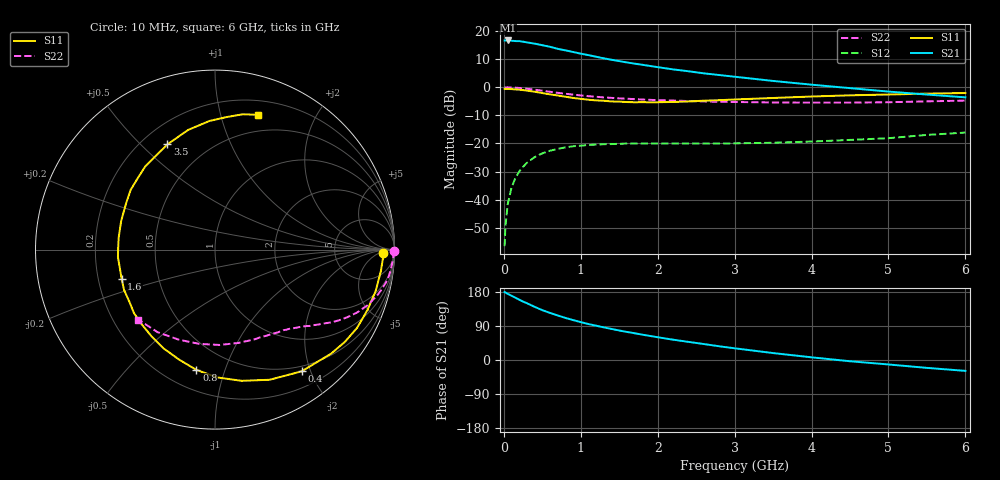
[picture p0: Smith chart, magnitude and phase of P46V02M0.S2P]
! SIEMENS Small Signal Semiconductors
! BFP182
! Si NPN RF Bipolar Junction Transistor in SOT143
! VCE = 6 V  IC = 2 mA
! Common Emitter S-Parameters:  March  1996
# GHz  S  MA  R  50
!  f  S11  S21  S12  S22
! GHz  MAG  ANG  MAG  ANG  MAG  ANG  MAG  ANG
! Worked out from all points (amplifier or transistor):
!   36 points, 10 MHz to 6 GHz, reference 50 ohm
!   highest |S21| = 16.6 dB at 50 MHz (marker M1)
!   |S21| within 3 dB of that: start of sweep to 704.2 MHz
!   unconditionally stable (mu >= 1): 2.231 GHz to 5.925 GHz
!   at 250 MHz: K = 0.12, MSG = 22.2 dB, |S12| = -28.3 dB
!   at 1.4 GHz: K = 0.66, MSG = 15.0 dB, |S12| = -20.2 dB
!   at 6 GHz: K = 0.99, MSG = 6.3 dB, |S12| = -16.1 dB
!   lowest NFmin = 1.10 dB at 450 MHz
!   S11 on the Smith chart (normalised r, x): 10 MHz: 27, -8; 400 MHz: 0.42, -1.86; 800 MHz: 0.32, -0.80; 1.6 GHz: 0.30, -0.14; 3.5 GHz: 0.30, +0.60; 6 GHz: 0.33, +1.32
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0.01  0.9351 -1.2  6.766 179.2  0.0015 88.4  0.9949 -0.5
0.02  0.9367 -3.2  6.755 178.4  0.0033 88.6  0.9911 -1.0
0.05  0.9318 -7.4  6.768 174.7  0.0083 88.7  0.9949 -2.8
0.1  0.9246 -14.4  6.694 169.6  0.0165 80.5  0.987 -5.6
0.15  0.9138 -21.5  6.6 164.4  0.0243 77.7  0.9807 -8.4
0.2  0.9039 -28.8  6.585 159.1  0.0318 73.6  0.97 -10.9
0.25  0.8877 -35.4  6.434 154.1  0.0386 69.8  0.9541 -13.5
0.4  0.8323 -54.6  5.942 140.2  0.0573 58.7  0.904 -20.1
0.5  0.7866 -67.2  5.577 131.6  0.0668 52.4  0.8657 -23.9
0.6  0.7461 -78.5  5.23 124.2  0.0744 47.0  0.8286 -27.0
0.8  0.6781 -98.8  4.515 111.1  0.0853 38.3  0.7663 -31.9
1  0.6205 -117.5  3.94 99.9  0.0916 31.6  0.7139 -35.7
1.1  0.5991 -126.1  3.715 94.8  0.0941 28.9  0.693 -37.4
1.3  0.5738 -141.8  3.262 86.1  0.0971 24.5  0.6594 -40.3
1.6  0.5449 -162.8  2.753 74.1  0.0998 19.6  0.6249 -44.3
1.8  0.5424 -175.6  2.504 66.8  0.0996 17.7  0.6049 -46.9
2.2  0.5467 162.9  2.072 53.6  0.1 14.8  0.5795 -52.7
2.8  0.5878 136.5  1.646 36.2  0.1003 13.9  0.5499 -62.5
3.5  0.6434 114.3  1.292 18.3  0.1032 14.6  0.5359 -76.1
4.5  0.7173 92.5  0.963 -3.3  0.1158 17.1  0.5325 -99.5
5.5  0.7696 78.4  0.741 -20.8  0.1421 17.9  0.5604 -124.8
6  0.7884 72.3  0.66 -28.7  0.1564 15.0  0.5781 -137.5
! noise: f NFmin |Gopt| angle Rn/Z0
0.45  1.1  0.42  29  0.36
0.9  1.2  0.4  58  0.3
1.8  1.85  0.32  126  0.22
